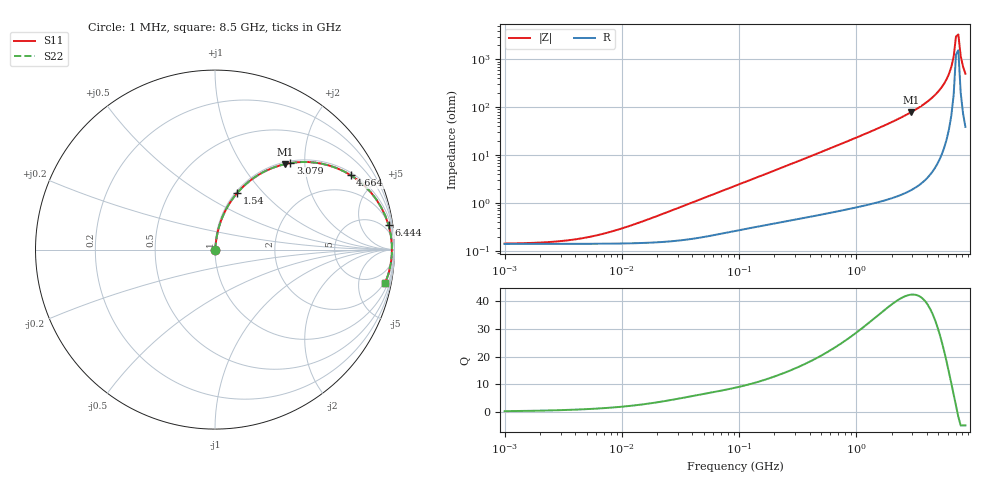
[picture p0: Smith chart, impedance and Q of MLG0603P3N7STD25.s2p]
! S-Parameter Data Generated by TDK Corporation
! Copyright(C) 2025 TDK Corporation.
! All Rights Reserved.
! TDK P/N: MLG0603P3N7STD25 (SMD / SMT Inductor (Coil))
! Property: L=3.7nH at 500MHz
! Size(LxWxT): 0.6x0.3x0.3mm
! Model Type: s2p (Touchstone File Format Version 1.0)
! Frequency: DC=Yes Start=1MHz Stop=8500MHz 198points Log-sweep
! Model Generated on Feb. 6, 2025
! Terms and conditions regarding TDK Simulation Models:
! 1)This simulation model is being provided solely for informational
!  purposes. Please refer to the specifications of the products in
!  terms of detailed characteristics of such products.
! 2)In no event shall TDK Corporation of any of its subsidiaries be
!  liable for any loss or damage arising, directly or indirectly,
!  from any information contained in this simulation model, including,
!  but not limited to loss or damages arising from any inaccuracies,
!  omissions or errors in connection with such information.
! 3)Any and all copyrights on this simulation model are owned by
!  TDK Corporation.  Duplication or redistribution of this simulation
!  model without prior written permission from TDK Corporation
!  is prohibited.
! 4)This simulation model is subject to any modification or change
!  without any prior notice.
! 5)Neither TDK Corporation nor any of its subsidiaries shall make any
!  warranty, express or implied, including but not limited to the
!  correctness, implied warranties of merchantability and fitness for
!  a particular purpose with respect to this simulation models.
! 6)The use of this simulation model shall be deemed to have consented
!  to the terms and conditions hereof.
! Port Assignments:
!  1 ---@@@--- 2
! Applicable Conditions:
!  Temperature = 25 degC
!  DC Bias Current = 0 A
!  Small Signal Operation
# Hz S MA R 50
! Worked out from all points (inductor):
!   197 points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, 1 MHz to 8.5 GHz, reference 50 ohm
!   read as one part in series: L = 4.09 nH near 17.5 MHz
!   highest Q = 42.5 at 2.94 GHz (marker M1), where L = 4.3 nH
!   self-resonance near 7.067 GHz
!   S11 on the Smith chart (normalised r, x): 1 MHz: 1.00, +0.00; 1.54 GHz: 1.02, +0.73; 3.079 GHz: 1.04, +1.69; 4.664 GHz: 1.11, +3.58; 6.444 GHz: 2, +14; 8.5 GHz: 2, -10
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1000000  0.001422 10.4  0.9986 -0.0  0.9986 -0.0  0.001422 10.4
2403882  0.001531 23.9  0.9986 -0.0  0.9986 -0.0  0.001531 23.9
4587603  0.001837 40.1  0.9986 -0.1  0.9986 -0.1  0.001837 40.1
9168677  0.002759 58.8  0.9986 -0.1  0.9986 -0.1  0.002759 58.8
2.10461e7  0.005611 74.0  0.9985 -0.3  0.9985 -0.3  0.005611 74.0
9.219544e7  0.02272 82.1  0.9971 -1.3  0.9971 -1.3  0.02272 82.1
4.229561e8  0.09775 81.3  0.99 -5.6  0.99 -5.6  0.09775 81.3
1.540426e9  0.3408 68.5  0.9305 -19.9  0.9305 -19.9  0.3408 68.5
1.940355e9  0.4235 63.5  0.895 -25.0  0.895 -25.0  0.4235 63.5
2.939772e9  0.6146 50.7  0.7745 -37.9  0.7745 -37.9  0.6146 50.7
3.07866e9  0.6389 49.0  0.7544 -39.7  0.7544 -39.7  0.6389 49.0
3.877948e9  0.7649 38.7  0.6253 -49.9  0.6253 -49.9  0.7649 38.7
4.664383e9  0.8622 28.8  0.4814 -59.5  0.4814 -59.5  0.8622 28.8
5.610304e9  0.9407 17.4  0.2988 -70.0  0.2988 -70.0  0.9407 17.4
6.152938e9  0.9673 11.2  0.1953 -74.8  0.1953 -74.8  0.9673 11.2
6.44363e9  0.9765 8.1  0.1413 -76.4  0.1413 -76.4  0.9765 8.1
6.748056e9  0.9827 4.9  0.08662 -76.0  0.08662 -76.0  0.9827 4.9
7.066863e9  0.9858 1.7  0.03279 -63.4  0.03279 -63.4  0.9858 1.7
7.400733e9  0.9857 -1.5  0.02974 60.5  0.02974 60.5  0.9857 -1.5
7.750377e9  0.9824 -4.7  0.08327 75.5  0.08327 75.5  0.9824 -4.7
8.116539e9  0.976 -7.9  0.138 76.1  0.138 76.1  0.976 -7.9
8.5e9  0.9666 -11.0  0.192 74.5  0.192 74.5  0.9666 -11.0
